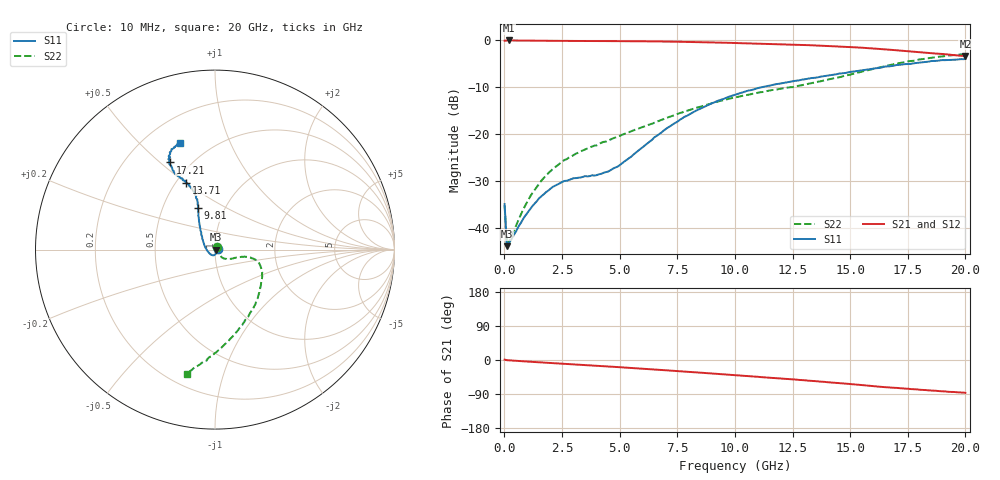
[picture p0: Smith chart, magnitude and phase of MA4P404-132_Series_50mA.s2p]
! AWR Design Environment (9226) Thu Aug 19 02:30:18 2021
! Document = '50mA'
! nPorts: 2, nXvals: 201
# GHz S DB R 50
!Freq DBS11 AngS11 DBS21 AngS21 DBS12 AngS12 DBS22 AngS22
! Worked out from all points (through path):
!   201 points, 10 MHz to 20 GHz, reference 50 ohm
!   highest |S21| = -0.11 dB at 210 MHz (marker M1); lowest = -3.4 dB at 20 GHz (marker M2)
!   group delay of S21, straight-line fit = 12.2 ps
!   lowest |S11| = -43.9 dB at 110 MHz (marker M3), VSWR 1.01, Z = 50.6 - j0.0766 ohm
!   |S11| at or under -10 dB: start of sweep to 11.22 GHz
!   |S22| runs from -43.9 to -3.0 dB; largest |S21 - S12| = 0.034
!   S11 on the Smith chart (normalised r, x): 10 MHz: 1.03, +0.01; 9.81 GHz: 0.75, +0.37; 13.71 GHz: 0.56, +0.50; 17.21 GHz: 0.39, +0.54; 20 GHz: 0.34, +0.67
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0.01  -34.96 17.0  -0.17 1.0  -0.16 0.7  -35.28 44.4
0.11  -43.93 -6.8  -0.11 -0.5  -0.10 -0.5  -43.94 -7.2
0.21  -43.22 -13.9  -0.11 -0.9  -0.10 -0.9  -42.81 -12.8
0.91  -37.44 -52.7  -0.14 -3.8  -0.13 -3.7  -35.24 -40.6
1.61  -33.29 -73.4  -0.17 -6.4  -0.16 -6.2  -29.95 -47.1
2.11  -31.28 -85.5  -0.19 -8.3  -0.18 -8.0  -27.43 -49.2
2.51  -30.23 -95.5  -0.20 -9.7  -0.19 -9.4  -25.91 -49.8
3.41  -29.16 -119.4  -0.23 -13.1  -0.21 -12.5  -23.53 -46.0
4.21  -28.51 -148.7  -0.24 -16.0  -0.22 -15.4  -21.90 -40.0
4.91  -27.00 -175.6  -0.26 -18.7  -0.24 -18.0  -20.59 -34.0
6.71  -20.10 136.6  -0.33 -25.9  -0.31 -25.0  -17.25 -18.1
7.81  -16.38 123.6  -0.41 -30.6  -0.41 -29.5  -15.23 -13.3
9.81  -12.00 112.4  -0.62 -39.1  -0.61 -37.6  -12.47 -14.5
10.01  -11.69 111.0  -0.65 -40.1  -0.63 -38.5  -12.26 -14.7
11.71  -9.51 109.9  -0.89 -47.5  -0.82 -45.7  -10.64 -26.7
13.41  -8.09 112.7  -1.16 -55.3  -1.06 -53.7  -9.10 -46.1
13.71  -7.83 113.1  -1.22 -57.0  -1.12 -55.1  -8.82 -50.0
14.81  -7.03 115.8  -1.46 -62.4  -1.35 -60.7  -7.58 -63.8
16.71  -5.63 117.9  -2.08 -72.6  -1.96 -70.9  -5.37 -85.2
17.21  -5.25 117.4  -2.28 -74.8  -2.17 -73.5  -4.86 -89.2
18.71  -4.46 114.8  -2.90 -81.2  -2.87 -80.7  -3.65 -98.6
20  -4.07 107.9  -3.43 -86.7  -3.53 -85.8  -2.99 -102.6
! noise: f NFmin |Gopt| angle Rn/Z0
0.01  0  1  0  2e-20
2.21  0  1  0  2e-20
4.41  0  1  0  2e-20
6.61  0  1  0  2e-20
8.81  0  1  0  2e-20
11.11  0  1  0  2e-20
13.31  0  1  0  2e-20
15.51  0  1  0  2e-20
17.71  0  1  0  2e-20
20  0  1  0  2e-20
